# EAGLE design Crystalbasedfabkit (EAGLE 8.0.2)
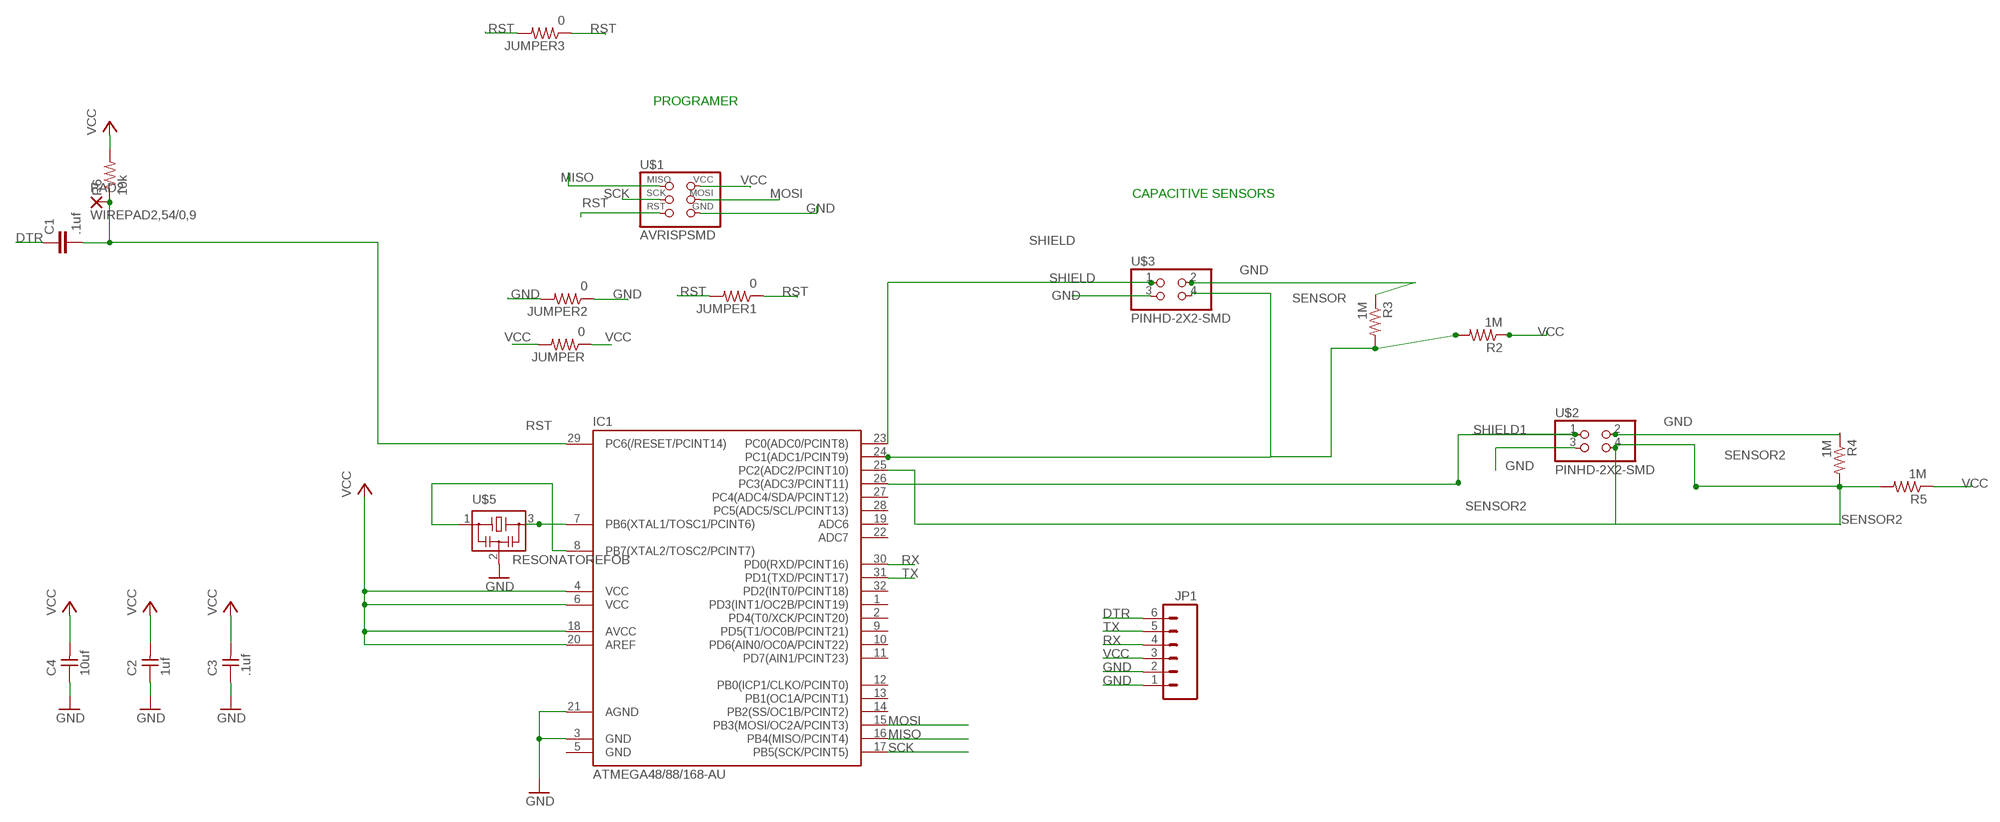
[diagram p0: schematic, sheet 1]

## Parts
C1  .1uf  C-EUC1206  [C1206]
C2  1uf  UNPOLARIZED_CAPACITOR1206  [1206]
C3  .1uf  UNPOLARIZED_CAPACITOR1206  [1206]
C4  10uf  UNPOLARIZED_CAPACITOR1206  [1206]
IC1  ATMEGA48/88/168-AU  [TQFP32-08]
JP1  M06SMD  [1X06-SMD]
JUMPER  0  RESISTOR1206  [1206]
JUMPER1  0  RESISTOR1206  [1206]
JUMPER2  0  RESISTOR1206  [1206]
JUMPER3  0  RESISTOR1206  [1206]
PAD2  WIREPAD2,54/0,9  [2,54/0,9]
R2  1M  RESISTOR1206  [1206]
R3  1M  RESISTOR1206  [1206]
R4  1M  RESISTOR1206  [1206]
R5  1M  RESISTOR1206  [1206]
R6  10k  RESISTOR1206  [1206]
U$1  AVRISPSMD  [2X03SMD]
U$2  PINHD-2X2-SMD  [2X02SMD]
U$3  PINHD-2X2-SMD  [2X02SMD]
U$5  RESONATOREFOB  [EFOBM]

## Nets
DTR: C1.1 JP1.6
GND: C2.1 C3.1 C4.1 IC1.3(GND) IC1.21(AGND) JP1.1 JP1.2 JUMPER2.1 JUMPER2.2 R3.1 R4.1 U$1.6(GND) U$2.2 U$2.3 U$3.2 U$3.3 U$5.2
MISO: IC1.16(PB4(MISO/PCINT4)) U$1.1(MISO)
MOSI: IC1.15(PB3(MOSI/OC2A/PCINT3)) U$1.4(MOSI)
N$15: IC1.8(PB7(XTAL2/TOSC2/PCINT7)) U$5.1
N$16: IC1.7(PB6(XTAL1/TOSC1/PCINT6)) U$5.3
RST: C1.2 IC1.29(PC6(/RESET/PCINT14)) JUMPER1.1 JUMPER1.2 JUMPER3.1 JUMPER3.2 PAD2.1(P) R6.1 U$1.5(RST)
RX: IC1.30(PD0(RXD/PCINT16)) JP1.4
SCK: IC1.17(PB5(SCK/PCINT5)) U$1.3(SCK)
SENSOR: IC1.24(PC1(ADC1/PCINT9)) R2.2 R3.2 U$3.4
SENSOR2: IC1.25(PC2(ADC2/PCINT10)) R4.2 R5.2 U$2.4
SHIELD: IC1.23(PC0(ADC0/PCINT8)) U$3.1
SHIELD1: IC1.26(PC3(ADC3/PCINT11)) U$2.1
TX: IC1.31(PD1(TXD/PCINT17)) JP1.5
VCC: C2.2 C3.2 C4.2 IC1.4(VCC) IC1.6(VCC) IC1.18(AVCC) IC1.20(AREF) JP1.3 JUMPER.1 JUMPER.2 R2.1 R5.1 R6.2 U$1.2(VCC)
Unconnected: IC1.1(PD3(INT1/OC2B/PCINT19)) IC1.2(PD4(T0/XCK/PCINT20)) IC1.9(PD5(T1/OC0B/PCINT21)) IC1.10(PD6(AIN0/OC0A/PCINT22)) IC1.11(PD7(AIN1/PCINT23)) IC1.12(PB0(ICP1/CLKO/PCINT0)) IC1.13(PB1(OC1A/PCINT1)) IC1.14(PB2(SS/OC1B/PCINT2)) IC1.19(ADC6) IC1.22(ADC7) IC1.27(PC4(ADC4/SDA/PCINT12)) IC1.28(PC5(ADC5/SCL/PCINT13)) IC1.32(PD2(INT0/PCINT18))

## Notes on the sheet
- PROGRAMER
- CAPACITIVE SENSORS

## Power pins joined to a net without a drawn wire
GND: IC1.5(GND)

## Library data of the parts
C1 = rcl:C-EU: CAPACITOR, European symbol
C2-C4 = ng:UNPOLARIZED_CAPACITOR: unpolarized_capacitor
IC1 = atmega8:ATMEGA48/88/168
JP1 = SparkFun:M06: Header 6 Standard 6-pin 0.1" header. Use with straight break away headers (SKU : PRT-00116), right angle break away headers (PRT-00553), swiss pins (PRT-00743), machine pins (PRT-00117), and female headers (PRT-00115). Molex polarized connector foot print use with SKU : PRT-08094 with associated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
JUMPER JUMPER1-JUMPER3 R2-R6 = ng:RESISTOR
PAD2 = wirepad:WIREPAD: Wire PAD connect wire on PCB
U$1 = 01fab:AVRISP
U$2 U$3 = 01fab:PINHD-2X2-SMD
U$5 = fab:RESONATOR

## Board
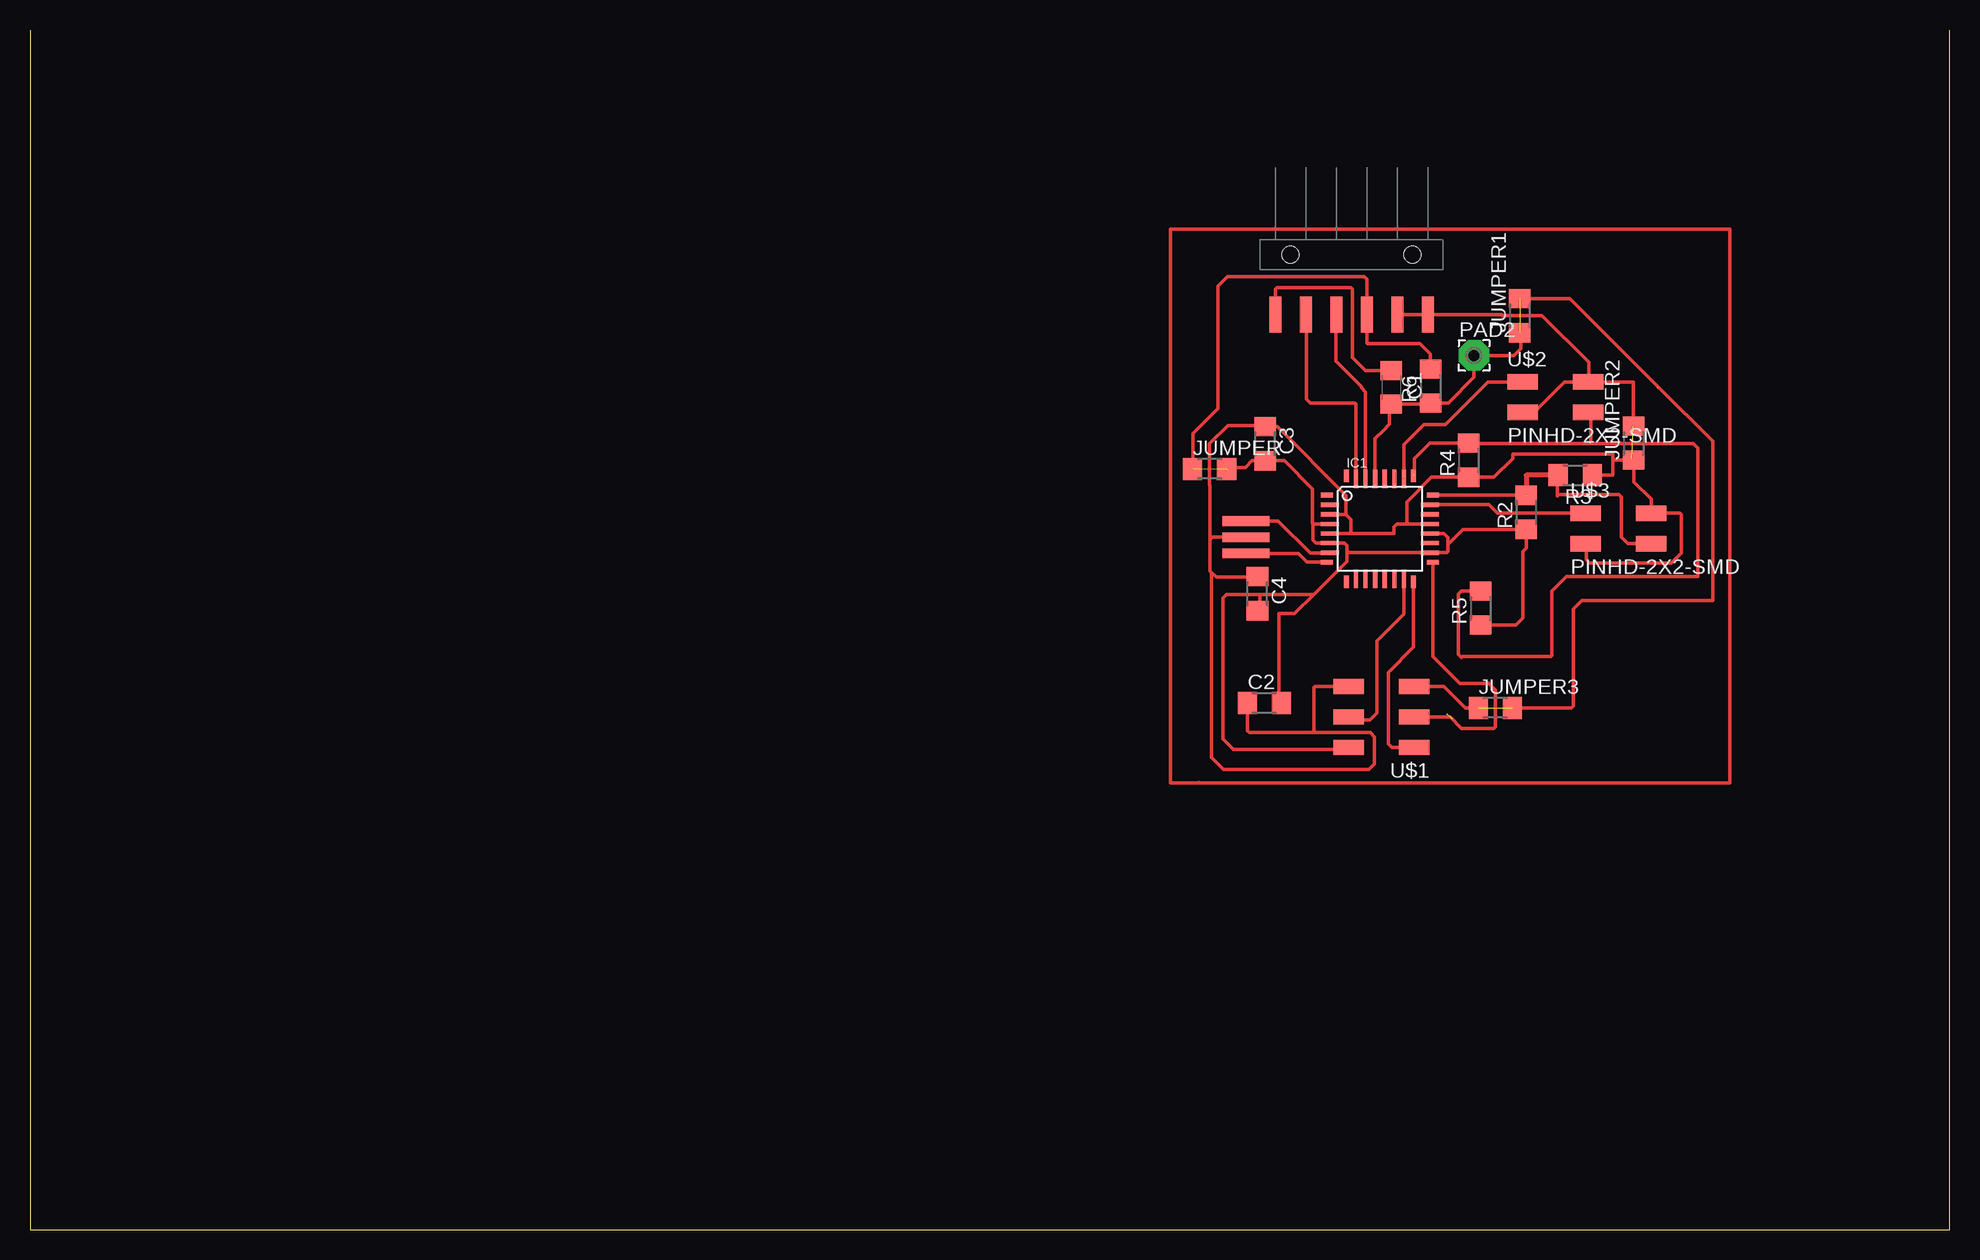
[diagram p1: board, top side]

Size 160 x 100 mm. Coordinates in mm from the lower left corner, seen from the top.
Outline: 160,100 160,0 0,0 0,100
Copper layers (1*16): Top 0.035mm / dielectric 1.5mm / Bottom 0.035mm
Design rules "default": minimum track width 0.4mm, minimum drill 0.4mm, track to track 0.4mm, track to pad 0.4mm, pad to pad 0.4mm, via to via 0.4mm, smd to smd 0.4mm, copper to edge 0.4mm, drill to drill 0.4mm, minimum pad ring 10mil, minimum via ring 8mil, stop-mask expansion 4mil, vias tented up to drill 0mil, thermal gap 10mil

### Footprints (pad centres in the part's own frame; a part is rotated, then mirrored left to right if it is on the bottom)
C1206 = smd 1.6 x 1.8: 1 -1.4,0; 2 1.4,0
1206 = smd 1.6 x 1.803: 1 -1.422,0; 2 1.422,0
TQFP32-08 = smd 1.016 x 0.406: 1 -4.42,2.8; 8 -4.42,-2.8; 17 4.42,-2.8; 24 4.42,2.8 | smd 1.524 x 0.356: 2 -4.166,2; 3 -4.166,1.2; 4 -4.166,0.4; 5 -4.166,-0.4; 6 -4.166,-1.2; 7 -4.166,-2; 18 4.166,-2; 19 4.166,-1.2; 20 4.166,-0.4; 21 4.166,0.4; 22 4.166,1.2; 23 4.166,2 | smd 0.406 x 1.016: 9 -2.8,-4.42; 16 2.8,-4.42; 25 2.8,4.42; 32 -2.8,4.42 | smd 0.356 x 1.524: 10 -2,-4.166; 11 -1.2,-4.166; 12 -0.4,-4.166; 13 0.4,-4.166; 14 1.2,-4.166; 15 2,-4.166; 26 2,4.166; 27 1.2,4.166; 28 0.4,4.166; 29 -0.4,4.166; 30 -1.2,4.166; 31 -2,4.166
1X06-SMD = smd 1 x 3: 1 -6.35,5; 2 -3.81,5; 3 -1.27,5; 4 1.27,5; 5 3.81,5; 6 6.35,5 | hole 1.4: -5.08,0; 5.08,0
2,54/0,9 = drill 0.914 pad 2.54 octagon: 1 0,0
2X03SMD = smd 2.54 x 1.27: 1 -2.54,2.54; 2 2.92,2.54; 3 -2.54,0; 4 2.92,0; 5 -2.54,-2.54; 6 2.92,-2.54
2X02SMD = smd 2.54 x 1.27: 1 -2.54,1.27; 2 2.92,1.27; 3 -2.54,-1.27; 4 2.92,-1.27
EFOBM = smd 0.8 x 3.9: 1 -1.35,0; 2 0,0; 3 1.35,0

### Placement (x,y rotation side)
C1  113.46,70.21 270 top
C2  102.9,43.89 0 top
C3  102.95,65.51 270 top
C4  102.31,53.01 270 top
IC1  112.52,58.42 0 top
JP1  110.16,81.25 180 top
JUMPER  98.32,63.4 0 top
JUMPER1  124.18,76.17 90 top
JUMPER2  133.65,65.56 90 top
JUMPER3  122.15,43.48 0 top
PAD2  120.37,72.87 0 top
R2  124.71,59.79 90 top
R3  128.8,62.89 180 top
R4  119.91,64.14 90 top
R5  120.9,51.82 90 top
R6  116.74,70.31 90 top
U$1  112.85,42.72 180 top
U$2  126.95,69.39 0 top
U$3  132.21,58.45 0 top
U$5  101.35,57.71 90 top

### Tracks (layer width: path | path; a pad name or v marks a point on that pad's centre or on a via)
DTR
  Top 0.305: C1.1 111.33,71.61 110.24,72.69 110.24,78.38 110.11,78.51 104.11,78.51 | 103.94,78.51 104.11,78.51 | 103.81,78.38 JP1.6 | 103.81,78.38 103.94,78.51 | 104.11,78.51 103.94,78.51 | 103.94,78.51 103.81,78.38
GND  (1 unrouted)
  Top 0.305: 108.38,59.64 IC1.3 109.67,59.62 | U$2.3 125.37,68.12 127.91,70.66 U$2.2 | 108.38,58.04 IC1.5 109.91,58.02 | 101.47,43.94 C2.1 101.5,43.87 101.5,41.55 101.62,41.43 107.04,41.43 | 109.91,58.02 113.69,58.02 113.69,58.57 113.94,58.82 114.73,58.82 | 114.73,58.82 IC1.21 | 109.67,59.62 110.08,59.21 110.08,58.2 109.91,58.02 | 109.67,59.62 109.7,59.65 109.7,61.19 103.96,66.93 103.45,66.93 | 103.45,66.93 C3.1 | 119.84,62.71 116.81,62.71 114.76,60.66 114.76,58.84 114.73,58.82 | 119.84,62.71 R4.1 | R4.1 | JUMPER2.2 133.66,70.66 U$2.2 | U$3.2 135.13,60.88 133.71,62.31 133.71,64.08 JUMPER2.1 | R4.1 122.02,62.71 123.6,64.29 123.6,64.64 131.93,64.64 131.93,64.14 | JUMPER2.1 133.5,64.29 133.5,64.14 JUMPER2.1 | R4.1 119.84,62.71 | U$2.2 129.92,70.72 129.92,72.31 126.03,76.2 122.73,76.2 122.68,76.25 JP1.1 | 116.67,76.1 JP1.1 | JP1.2 JP1.1 | 131.93,64.14 JUMPER2.1 | R3.1 131.93,62.89 131.93,64.14 | U$3.3 129.72,57.12 129.72,55.85 130,55.58 136.83,55.58 137.64,56.39 137.64,59.61 137.54,59.72 U$3.2 | 135.15,59.69 U$3.2 | 100.81,57.71 U$5.2 100.81,57.71 | 100.81,57.71 98.58,57.71 98.35,57.48 98.35,57.28 | 98.35,57.28 98.35,54.91 98.48,54.79 | 98.48,54.79 98.88,54.38 102.26,54.38 C4.1 | 98.48,54.79 98.48,39.37 99.49,38.35 111.61,38.35 112.06,38.81 112.06,41.07 111.71,41.43 107.04,41.43 | U$1.6 107.09,45.26 107.01,45.19 107.01,41.45 107.04,41.43 | 98.35,57.28 98.35,62.03 98.32,62.05 98.32,65.51 99.85,67.03 103.35,67.03 103.45,66.93
  Top 0.406: 130.5,62.89 R3.1
MISO
  Top 0.305: IC1.16 115.32,48.55 113.23,46.46 113.23,40.49 113.54,40.18 U$1.1
MOSI
  Top 0.305: IC1.15 114.52,51.33 112.27,49.07 112.27,48.08 | 108.89,42.7 108.84,42.65 109.86,42.65 U$1.4 110.16,42.49 111.68,42.49 112.27,43.08 112.27,48.08 | 112.27,48.08 112.27,47.88
N$1
  Top 0.305: 96.44,37.24 141.68,37.24 141.68,83.39 95.05,83.39 95.05,37.24 97.43,37.24 97.43,37.29
N$15
  Top 0.305: U$5.1 105.72,56.36 106.43,55.65 108.07,55.65 IC1.8
N$16
  Top 0.305: 102.54,59.06 104.04,59.06 106.71,56.39 107.16,56.39 107.42,56.39 108.32,56.39 IC1.7 | 102.54,59.06 U$5.3 102.54,59.06
RST  (3 unrouted)
  Top 0.305: IC1.29 112.12,65.92 112.8,66.6 112.8,66.62 113.31,67.13 113.31,68.65 C1.2 116.66,68.81 R6.1 116.76,68.91 118.21,68.91 120.37,71.07 120.37,72.64 PAD2.1 123.7,72.87 124.26,73.43 124.26,74.68 JUMPER1.1 | 135.76,70.21 135.71,70.21 | 135.76,70.21 140.26,65.71 140.26,52.43 129.34,52.43 128.65,51.74 128.65,43.66 128.47,43.48 128.32,43.48 127.51,43.48 JUMPER3.2 | JUMPER1.2 128.37,77.6 135.76,70.21 | JUMPER3.1 119.63,43.48 117.86,45.26 U$1.5
RX
  Top 0.305: IC1.30 111.32,69.83 110.97,70.18 110.97,70.26 108.84,72.39 108.84,76.2 JP1.4
SCK  (2 unrouted)
  Top 0.305: 115.49,42.82 U$1.3 118.39,42.72 119.33,41.78 122.02,41.78 122.15,41.91 122.15,44.98 121.61,45.52 119.2,45.52 116.94,47.78 IC1.17
SENSOR  (1 unrouted)
  Top 0.305: 135.05,57.1 U$3.4 133.17,57.17 132.64,57.71 132.64,61.06 132.44,61.27 127.43,61.27 127.33,61.16 127.33,62.84 R3.2 | IC1.24 R2.2
  Top 0.406: R3.2 124.71,62.89 R2.2
SENSOR2  (3 unrouted)
  Top 0.305: R5.2 119.33,53.24 119.08,52.98 119.08,47.95 119.33,47.7 119.38,47.75 126.77,47.75 126.87,47.85 126.87,53.24 128.07,54.43 139.01,54.43 139.01,65.15 138.66,65.51 130.1,65.51 | R4.2 120.02,65.66 120.02,65.56 R4.2 | 119.96,65.51 130.1,65.51 | 119.96,65.51 R4.2 | 130.1,65.51 130.1,67.89 U$2.4 | R4.2 119.96,65.56 119.96,65.51 | IC1.25 115.37,62.88 | R4.2 116.69,65.56 115.39,64.26 115.39,62.91
SHIELD
  Top 0.305: IC1.23 121.62,60.42 122.3,59.74 130.18,59.74 130.25,59.66 129.72,59.66 U$3.1
SHIELD1  (1 unrouted)
  Top 0.305: IC1.26 114.52,65.42 116.2,67.11 117.98,67.11 121.54,70.66 U$2.1
TX
  Top 0.305: IC1.31 110.52,68.8 110.44,68.89 106.73,68.89 106.38,69.24 106.38,76.23 JP1.5
VCC  (2 unrouted)
  Top 0.305: 109.78,56.59 109.78,57.02 109.58,57.23 IC1.6 107.19,57.22 106.93,57.48 106.93,58.81 106.94,58.82 | 109.78,56.59 109.78,55.7 107.02,52.95 | 107.02,52.95 105.41,51.33 104.09,51.33 104.09,44.12 C2.2 | 109.53,40.18 U$1.2 109.75,40.01 100.33,40.01 99.44,40.89 99.44,52.65 99.73,52.95 102.51,52.95 | R2.1 124.94,58.14 124.71,57.91 | 102.57,51.33 C4.2 102.51,51.79 102.51,52.95 | 107.02,52.95 102.51,52.95 | 109.78,56.59 109.95,56.42 IC1.18 116.71,56.44 118.11,56.44 118.19,56.52 118.19,57.12 | IC1.20 117.85,58.02 118.19,57.68 118.19,57.12 | R2.1 124.71,57.91 | R5.1 123.85,50.39 124.44,50.98 124.44,56.54 124.71,56.82 124.71,57.91 | 100.36,62.76 99.8,63.32 | JUMPER.2 99.87,63.52 101.3,63.52 101.85,64.08 C3.2 104.55,64.08 106.88,61.75 106.88,58.88 106.94,58.82 | JUMPER.1 96.95,63.45 96.95,66.34 99.03,68.43 99.03,78.64 99.82,79.43 111.23,79.43 111.43,79.22 JP1.3 111.43,73.91 111.48,73.86 115.85,73.86 116.74,72.97 R6.2 | 106.94,58.82 IC1.4 | R2.1 119.43,58.37 118.19,57.12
